(* Logix 5000 AddOnInstructionDefinition export Banner_B25_B55_Param_v4; software revision 33.00 *)

TYPE Banner_B25_B55_Configuration_v4 :
STRUCT
   Sensor_Lockout : SINT;   // 0=Unlocked, 1=Locked
   Sensitivity : SINT;   // 0=Low, 1=Standard, 2=High
   Pin2_Function : SINT;   // 0=Disabled, 1=Remote Teach, 2=Detection Output, 3=Complementary Output, 4=NC Health, 5=NO Health
   Pin2_Pin4_Polarity : SINT;   // 0=NPN, 1=PNP, 2=Push Pull
   Output_Logic : SINT;   // 0=LO, 1= DO
   Output_Delay_Mode : SINT;   // 0=No Delay, 1=On/Off Delay
   Output_On_Delay : DINT;
   Output_Off_Delay : DINT;
   Dynamic_Teach_Timeout_Mode : SINT;   // 0=Cancel Teach, 1=Stop Teach
   Dynamic_Teach_Timeout_Duration : DINT;
   Alarm_Threshold : SINT;   // Set to 0% to disable alarm. Thresholds close to 100% will alarm near taught condition, thrsholds near 0% will alarm near sensor limits
   Display_Disable : SINT;   // 0=Enabled, 1=Disabled
   Drift_Filter_Enable : SINT;   // 0=Disabled, 1=Enabled
   Signal_Mode : SINT;   // Signal Mode - Signal places 100% at taught condition and 0% at no signal. Switchpoint Centric paces 100% at taught conditition and 50% at switchpoint.
END_STRUCT
END_TYPE

TYPE Banner_B25_B55_RD_v4 :   // UDT that stores the Read Data for a B25 or B55.
STRUCT
   Direct : Banner_Direct_Parameters_v4;
   Serial_Number : STRING;
   Teach_State : SINT;   // 0=Idle, 1=SP1 Success, 2=SP2 Succes, 3=SP1 SP2 Success, 4 = Wait for Command, 5 = Busy, 7 = Error.
   Status : Banner_B25_B55_Status_v4;
   All_Time_Run_Time_Counter : DINT;   // 0 to 2 Billion. 1/4 hr increments.
END_STRUCT
END_TYPE

TYPE Banner_B25_B55_Status_v4 :
STRUCT
   Output_State : SINT;   // 0=Inactive, 1=Active
   Signal_Level : SINT;   // Signal Level - Switchpoit is at 50%, Taught Signal is at 100%
   Temperature : DINT;   // Internal Temperature
   Last_Taught_Temperature : DINT;   // Internal Temperature the last time device was taught
   Quality_of_Teach : SINT;   // 0=Not Taught, 1=Good, 2=Bad
   Health_Alarm_State : SINT;   // 0=No Alarm, 1= Alarm
   Quality_of_Health : INT;
END_STRUCT
END_TYPE

TYPE Banner_B25_B55_v4 :   // All of the parameters for a B25 or B55.
STRUCT
   Initial_Global_Read : BOOL;   // Determines if all of the IO-Link data has been read into the PLC yet
   Command : INT;   // Value placed in here will activate a read or write to a specifc IO-Link Index
   Read : Banner_B25_B55_RD_v4;   // Read Only Data
   Write : Banner_B25_B55_WD_v4;   // Write Data
   Reset : BOOL;   // Resets AOI. This will force a complete parameter read of the sensor.
END_STRUCT
END_TYPE

TYPE Banner_B25_B55_WD_v4 :   // UDT that stores the Write Data for a B25 or B55.
STRUCT
   System_Command : INT;   // See IODD file for list of commands that can be activated via the System Command interface
   Parameter_Access_Lock : SINT;   // Write access to all parameters is prohibited while value is 1. Only this parameter can be adjusted when value is 1.
   Data_Storage_Lock : SINT;   // Automatic data storage is disabled when this value is equal to 1. Read access is not affected.
   Local_Parameterization_Lock : SINT;   // Parameterization via local control elements on device is disabled.
   Local_User_Interface_Lock : SINT;   // Operation of local user interface is disabled.
   Configuration : Banner_B25_B55_Configuration_v4;
   Resettable_Run_Time_Counter : DINT;   // 0 to 2 Billion. 1/4 hr increments.
   All_Time_Run_Time_Event_Time : DINT;   // 0 to 2 Billion. 1/4 hr increments.
   Resettable_Run_Time_Event_Time_Counter : DINT;   // 0 to 2 Billion. 1/4 hr increments.
END_STRUCT
END_TYPE

TYPE Banner_Direct_Parameters_v4 :
STRUCT
   Master_Cycle_Time : INT;
   Min_Cycle_Time : INT;
   M_Sequence_Capability : INT;
   IO_Link_Version_ID : INT;
   Process_Data_Input_Length : INT;
   Process_Data_Output_Length : INT;
   Combined_Vendor_ID : DINT;   // IO-Link Vendor ID
   Vendor_ID1 : INT;
   Vendor_ID2 : INT;
   Combined_Device_ID : DINT;   // IO-Link Device ID
   Device_ID1 : INT;
   Device_ID2 : INT;
   Device_ID3 : INT;
END_STRUCT
END_TYPE

TYPE Banner_IOL_Port_v4 :   // UDT that has all of the data items necessary to communicate with a specific Port on a IO-Link Master
STRUCT
   Port_Controlled : INT;   // Each bit represents a port on an IO-Link Master. Set to 1 to tell AOI to control that port.
   Port_Activate : INT;   // Each bit represents a port on an IO-Link Master. When ON that port will process any commands in queue.
   Port_Read : INT;   // Each bit represents a port on an IO-Link Master. Used to determine when device AOI has requested a Read command.
   Port_Write : INT;   // Each bit represents a port on an IO-Link Master. Used to determine when device AOI has requested a Write command.
   Port_RW_Complete : INT;   // Each bit represents a port on an IO-Link Master. Tells device AOI that Read or Write request has been completed.
   Port_Device_Read : INT;
   Data_Transfer : SINT[190];   // Array to transfer data from IO-Master to device AOIs.
END_STRUCT
END_TYPE

ADD_ON_INSTRUCTION Banner_B25_B55_Param_v4   (* revision 4.0, vendor Banner Engineering *)
// AOI to read and write parameter data to an IO-Link B25 or B55.
VAR_IN_OUT
   Device : Banner_B25_B55_v4; {required}
   Port_Data : Banner_IOL_Port_v4; {required}
END_VAR
VAR_INPUT
   Port : DINT; {required}
   Type : DINT; {required}
END_VAR
VAR
   Local_Control : DINT; {access None}
   Global_Read_Command_Value : INT; {access None}
   Global_Write_Command_Value : INT; {access None}
   Command_Being_Processed : BOOL; {access None}
   Update_Archive : BOOL; {access None}
   Index_Write_Inprocess : INT; {access None}
   Index_Write_Control : INT; {access None}
   Inprocess_Index : DINT; {access None}
END_VAR

ROUTINE Logic   (* ladder *)
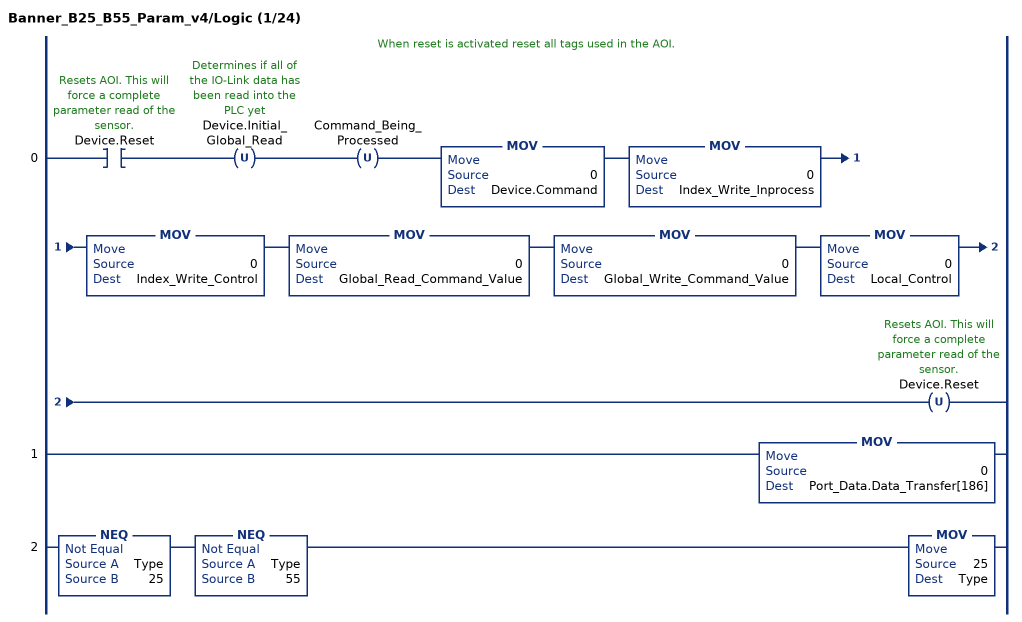
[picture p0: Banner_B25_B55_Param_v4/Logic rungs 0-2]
   // When reset is activated reset all tags used in the AOI.
   0: XIC(Device.Reset)OTU(Device.Initial_Global_Read)OTU(Command_Being_Processed)MOV(0,Device.Command)MOV(0,Index_Write_Inprocess)MOV(0,Index_Write_Control)MOV(0,Global_Read_Command_Value)MOV(0,Global_Write_Command_Value)MOV(0,Local_Control)OTU(Device.Reset);
   1: MOV(0,Port_Data.Data_Transfer[186]);
   2: NEQ(Type,25)NEQ(Type,55)MOV(25,Type);
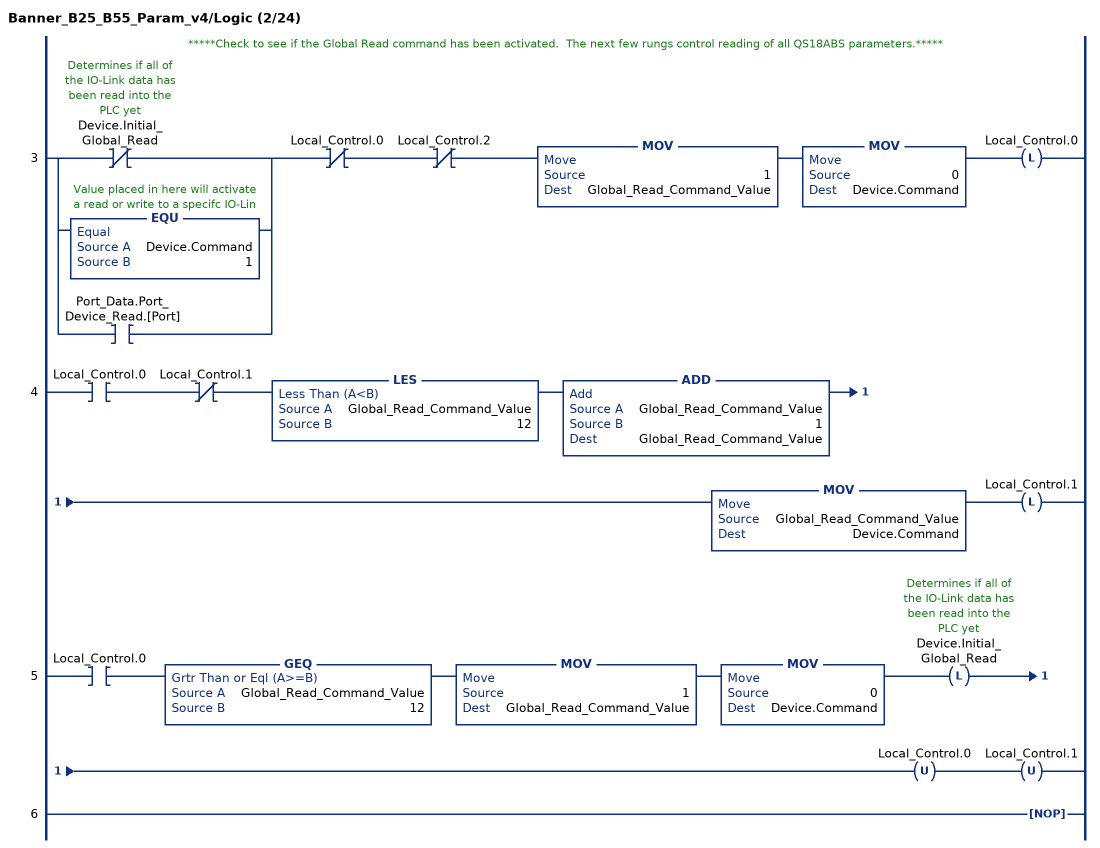
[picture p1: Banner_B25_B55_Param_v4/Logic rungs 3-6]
   // *****Check to see if the Global Read command has been activated.  The next few rungs control reading of all QS18ABS parameters.*****
   3: [XIO(Device.Initial_Global_Read) ,EQU(Device.Command,1) ,XIC(Port_Data.Port_Device_Read.[Port]) ]XIO(Local_Control.0)XIO(Local_Control.2)MOV(1,Global_Read_Command_Value)MOV(0,Device.Command)OTL(Local_Control.0);
   4: XIC(Local_Control.0)XIO(Local_Control.1)LES(Global_Read_Command_Value,12)ADD(Global_Read_Command_Value,1,Global_Read_Command_Value)MOV(Global_Read_Command_Value,Device.Command)OTL(Local_Control.1);
   5: XIC(Local_Control.0)GEQ(Global_Read_Command_Value,12)MOV(1,Global_Read_Command_Value)MOV(0,Device.Command)OTL(Device.Initial_Global_Read)OTU(Local_Control.0)OTU(Local_Control.1);
   6: NOP();
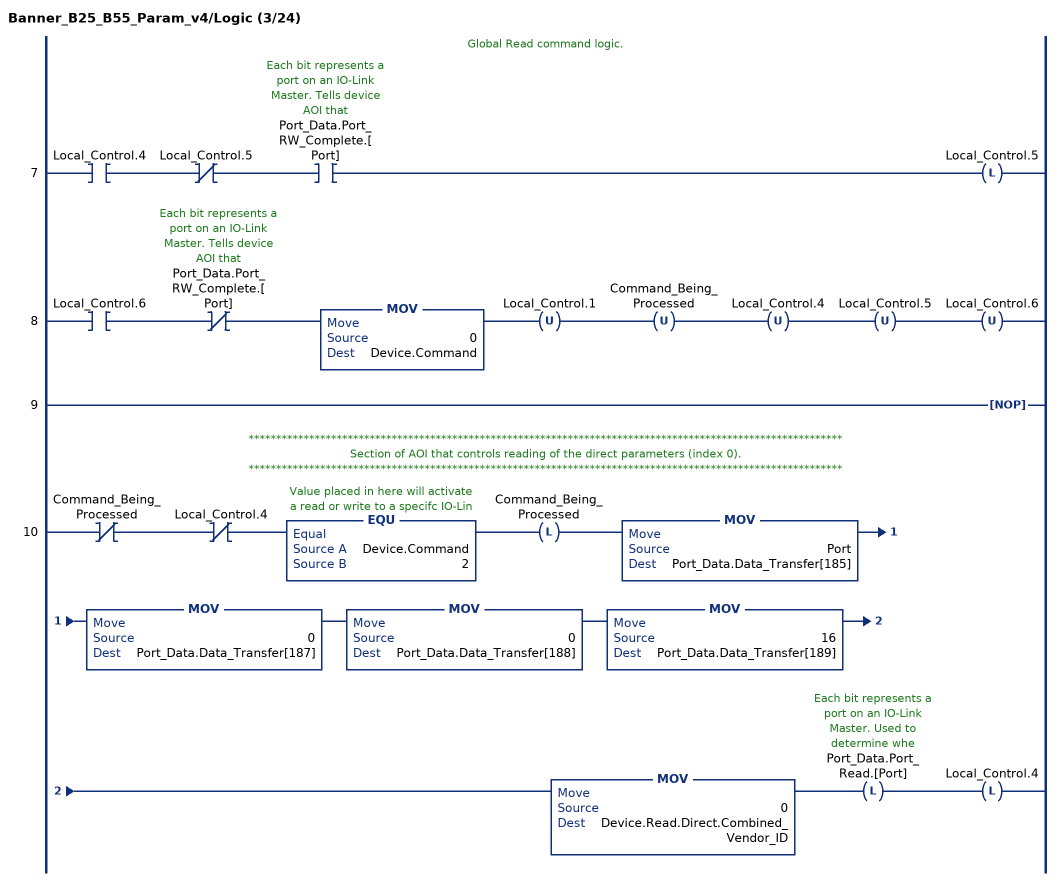
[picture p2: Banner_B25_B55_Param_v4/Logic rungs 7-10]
   // Global Read command logic.
   7: XIC(Local_Control.4)XIO(Local_Control.5)XIC(Port_Data.Port_RW_Complete.[Port])OTL(Local_Control.5);
   8: XIC(Local_Control.6)XIO(Port_Data.Port_RW_Complete.[Port])MOV(0,Device.Command)OTU(Local_Control.1)OTU(Command_Being_Processed)OTU(Local_Control.4)OTU(Local_Control.5)OTU(Local_Control.6);
   9: NOP();
   // ************************************************************************************************************
   // Section of AOI that controls reading of the direct parameters (index 0).
   // ************************************************************************************************************
   10: XIO(Command_Being_Processed)XIO(Local_Control.4)EQU(Device.Command,2)OTL(Command_Being_Processed)MOV(Port,Port_Data.Data_Transfer[185])MOV(0,Port_Data.Data_Transfer[187])MOV(0,Port_Data.Data_Transfer[188])MOV(16,Port_Data.Data_Transfer[189])MOV(0,Device.Read.Direct.Combined_Vendor_ID)OTL(Port_Data.Port_Read.[Port])OTL(Local_Control.4);
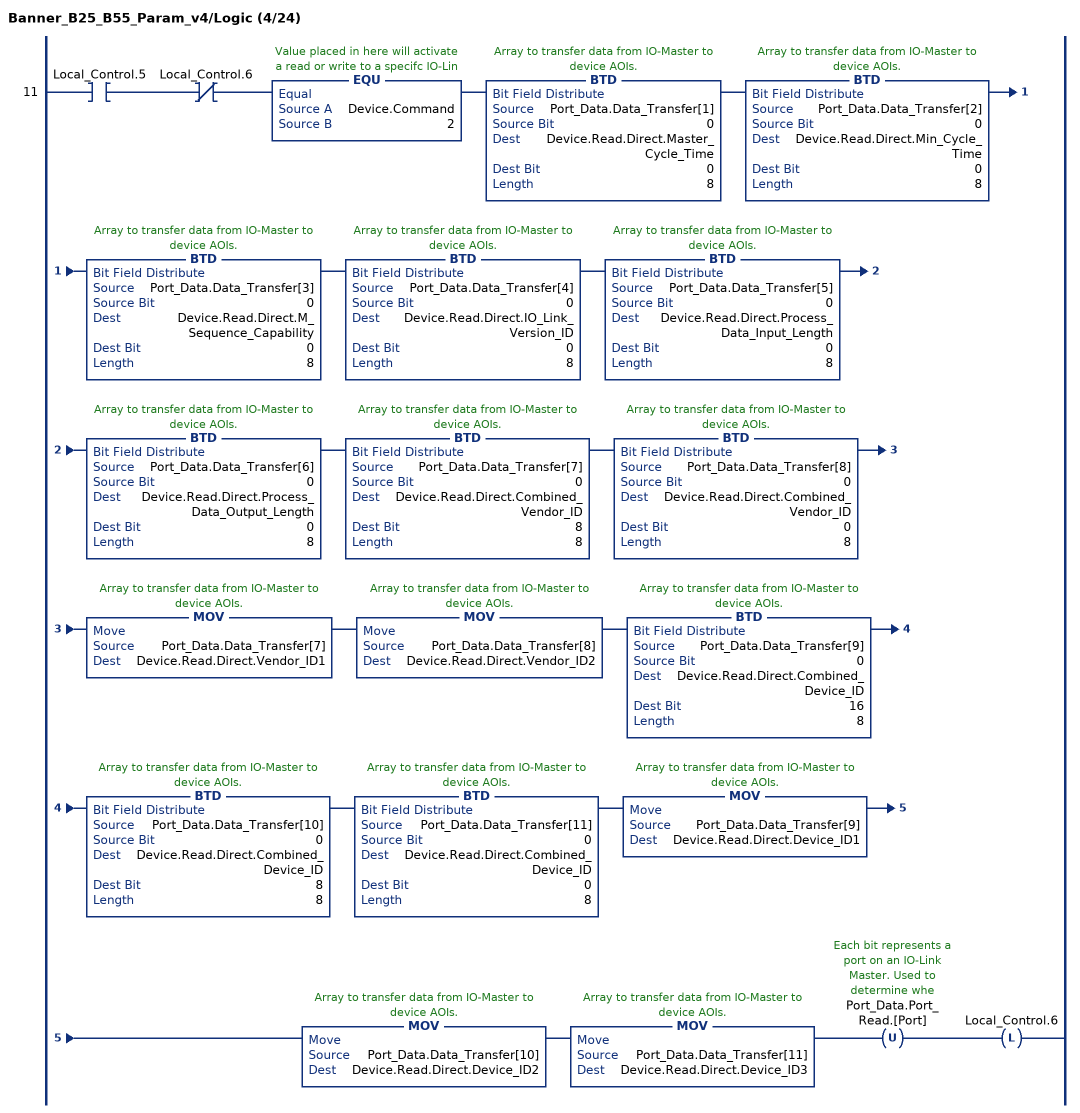
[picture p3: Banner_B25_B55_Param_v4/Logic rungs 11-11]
   11: XIC(Local_Control.5)XIO(Local_Control.6)EQU(Device.Command,2)BTD(Port_Data.Data_Transfer[1],0,Device.Read.Direct.Master_Cycle_Time,0,8)BTD(Port_Data.Data_Transfer[2],0,Device.Read.Direct.Min_Cycle_Time,0,8)BTD(Port_Data.Data_Transfer[3],0,Device.Read.Direct.M_Sequence_Capability,0,8)BTD(Port_Data.Data_Transfer[4],0,Device.Read.Direct.IO_Link_Version_ID,0,8)BTD(Port_Data.Data_Transfer[5],0,Device.Read.Direct.Process_Data_Input_Length,0,8)BTD(Port_Data.Data_Transfer[6],0,Device.Read.Direct.Process_Data_Output_Length,0,8)BTD(Port_Data.Data_Transfer[7],0,Device.Read.Direct.Combined_Vendor_ID,8,8)BTD(Port_Data.Data_Transfer[8],0,Device.Read.Direct.Combined_Vendor_ID,0,8)MOV(Port_Data.Data_Transfer[7],Device.Read.Direct.Vendor_ID1)MOV(Port_Data.Data_Transfer[8],Device.Read.Direct.Vendor_ID2)BTD(Port_Data.Data_Transfer[9],0,Device.Read.Direct.Combined_Device_ID,16,8)BTD(Port_Data.Data_Transfer[10],0,Device.Read.Direct.Combined_Device_ID,8,8)BTD(Port_Data.Data_Transfer[11],0,Device.Read.Direct.Combined_Device_ID,0,8)MOV(Port_Data.Data_Transfer[9],Device.Read.Direct.Device_ID1)MOV(Port_Data.Data_Transfer[10],Device.Read.Direct.Device_ID2)MOV(Port_Data.Data_Transfer[11],Device.Read.Direct.Device_ID3)OTU(Port_Data.Port_Read.[Port])OTL(Local_Control.6);
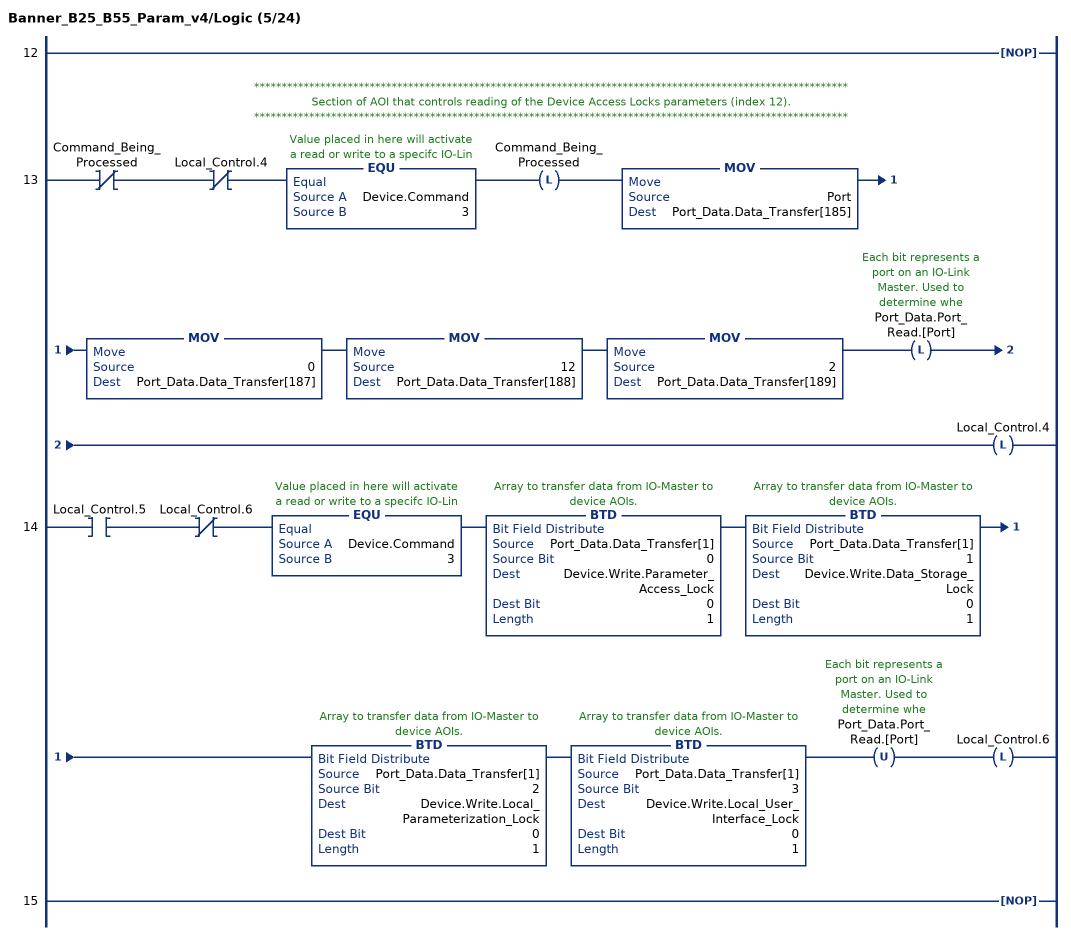
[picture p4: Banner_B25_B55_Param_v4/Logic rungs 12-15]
   12: NOP();
   // ************************************************************************************************************
   // Section of AOI that controls reading of the Device Access Locks parameters (index 12).
   // ************************************************************************************************************
   13: XIO(Command_Being_Processed)XIO(Local_Control.4)EQU(Device.Command,3)OTL(Command_Being_Processed)MOV(Port,Port_Data.Data_Transfer[185])MOV(0,Port_Data.Data_Transfer[187])MOV(12,Port_Data.Data_Transfer[188])MOV(2,Port_Data.Data_Transfer[189])OTL(Port_Data.Port_Read.[Port])OTL(Local_Control.4);
   14: XIC(Local_Control.5)XIO(Local_Control.6)EQU(Device.Command,3)BTD(Port_Data.Data_Transfer[1],0,Device.Write.Parameter_Access_Lock,0,1)BTD(Port_Data.Data_Transfer[1],1,Device.Write.Data_Storage_Lock,0,1)BTD(Port_Data.Data_Transfer[1],2,Device.Write.Local_Parameterization_Lock,0,1)BTD(Port_Data.Data_Transfer[1],3,Device.Write.Local_User_Interface_Lock,0,1)OTU(Port_Data.Port_Read.[Port])OTL(Local_Control.6);
   15: NOP();
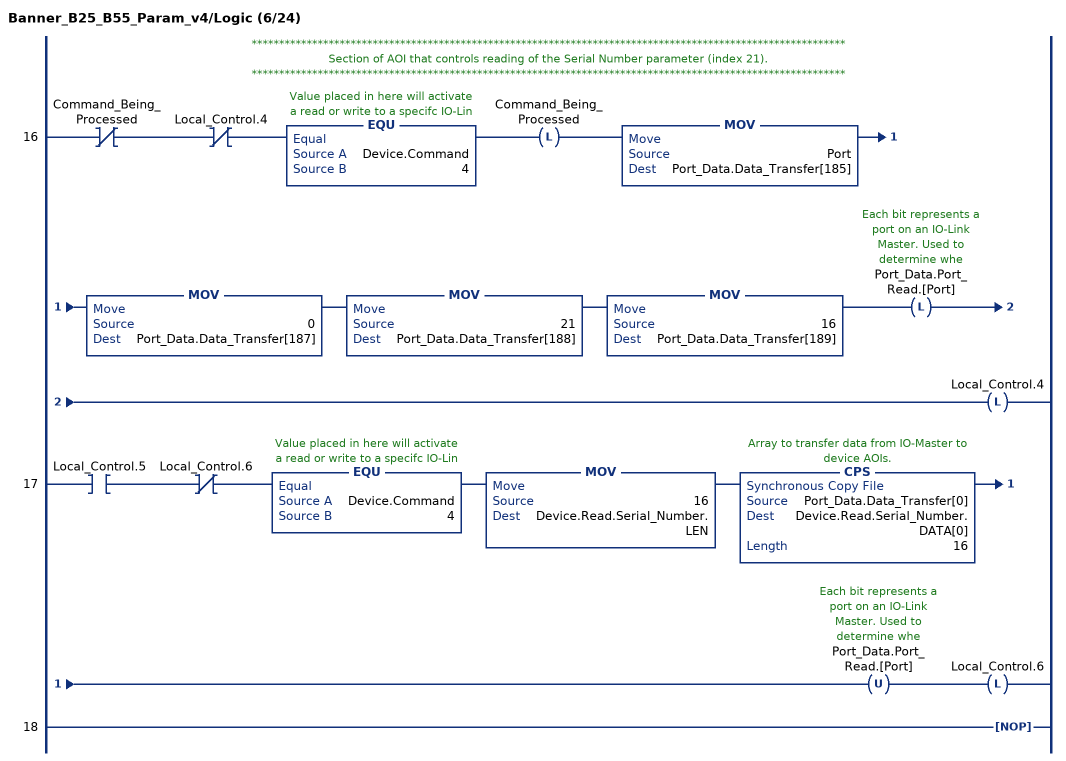
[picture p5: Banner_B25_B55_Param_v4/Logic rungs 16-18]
   // ************************************************************************************************************
   // Section of AOI that controls reading of the Serial Number parameter (index 21).
   // ************************************************************************************************************
   16: XIO(Command_Being_Processed)XIO(Local_Control.4)EQU(Device.Command,4)OTL(Command_Being_Processed)MOV(Port,Port_Data.Data_Transfer[185])MOV(0,Port_Data.Data_Transfer[187])MOV(21,Port_Data.Data_Transfer[188])MOV(16,Port_Data.Data_Transfer[189])OTL(Port_Data.Port_Read.[Port])OTL(Local_Control.4);
   17: XIC(Local_Control.5)XIO(Local_Control.6)EQU(Device.Command,4)MOV(16,Device.Read.Serial_Number.LEN)CPS(Port_Data.Data_Transfer[0],Device.Read.Serial_Number.DATA[0],16)OTU(Port_Data.Port_Read.[Port])OTL(Local_Control.6);
   18: NOP();
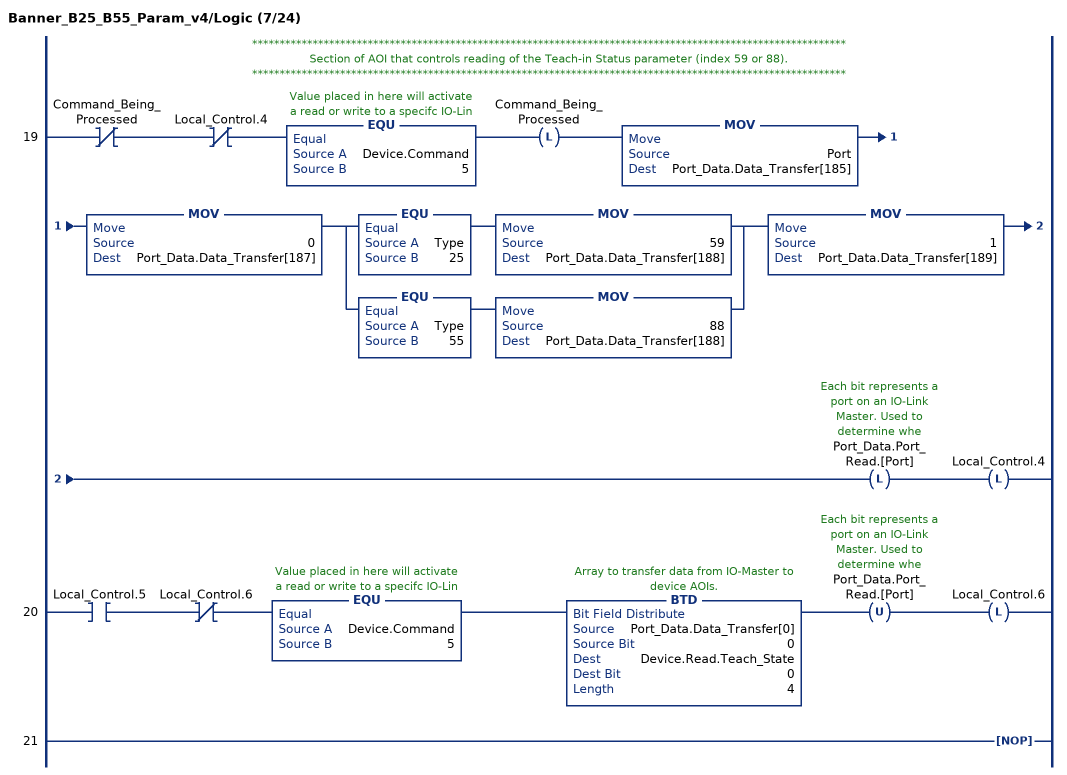
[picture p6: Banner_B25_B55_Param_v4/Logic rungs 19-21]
   // ************************************************************************************************************
   // Section of AOI that controls reading of the Teach-in Status parameter (index 59 or 88).
   // ************************************************************************************************************
   19: XIO(Command_Being_Processed)XIO(Local_Control.4)EQU(Device.Command,5)OTL(Command_Being_Processed)MOV(Port,Port_Data.Data_Transfer[185])MOV(0,Port_Data.Data_Transfer[187])[EQU(Type,25) MOV(59,Port_Data.Data_Transfer[188]) ,EQU(Type,55) MOV(88,Port_Data.Data_Transfer[188]) ]MOV(1,Port_Data.Data_Transfer[189])OTL(Port_Data.Port_Read.[Port])OTL(Local_Control.4);
   20: XIC(Local_Control.5)XIO(Local_Control.6)EQU(Device.Command,5)BTD(Port_Data.Data_Transfer[0],0,Device.Read.Teach_State,0,4)OTU(Port_Data.Port_Read.[Port])OTL(Local_Control.6);
   21: NOP();
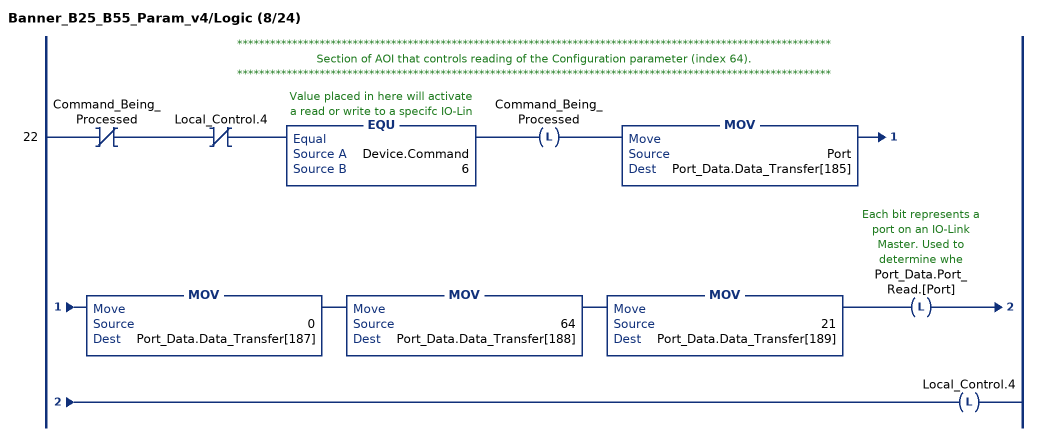
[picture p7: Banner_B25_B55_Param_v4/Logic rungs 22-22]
   // ************************************************************************************************************
   // Section of AOI that controls reading of the Configuration parameter (index 64).
   // ************************************************************************************************************
   22: XIO(Command_Being_Processed)XIO(Local_Control.4)EQU(Device.Command,6)OTL(Command_Being_Processed)MOV(Port,Port_Data.Data_Transfer[185])MOV(0,Port_Data.Data_Transfer[187])MOV(64,Port_Data.Data_Transfer[188])MOV(21,Port_Data.Data_Transfer[189])OTL(Port_Data.Port_Read.[Port])OTL(Local_Control.4);
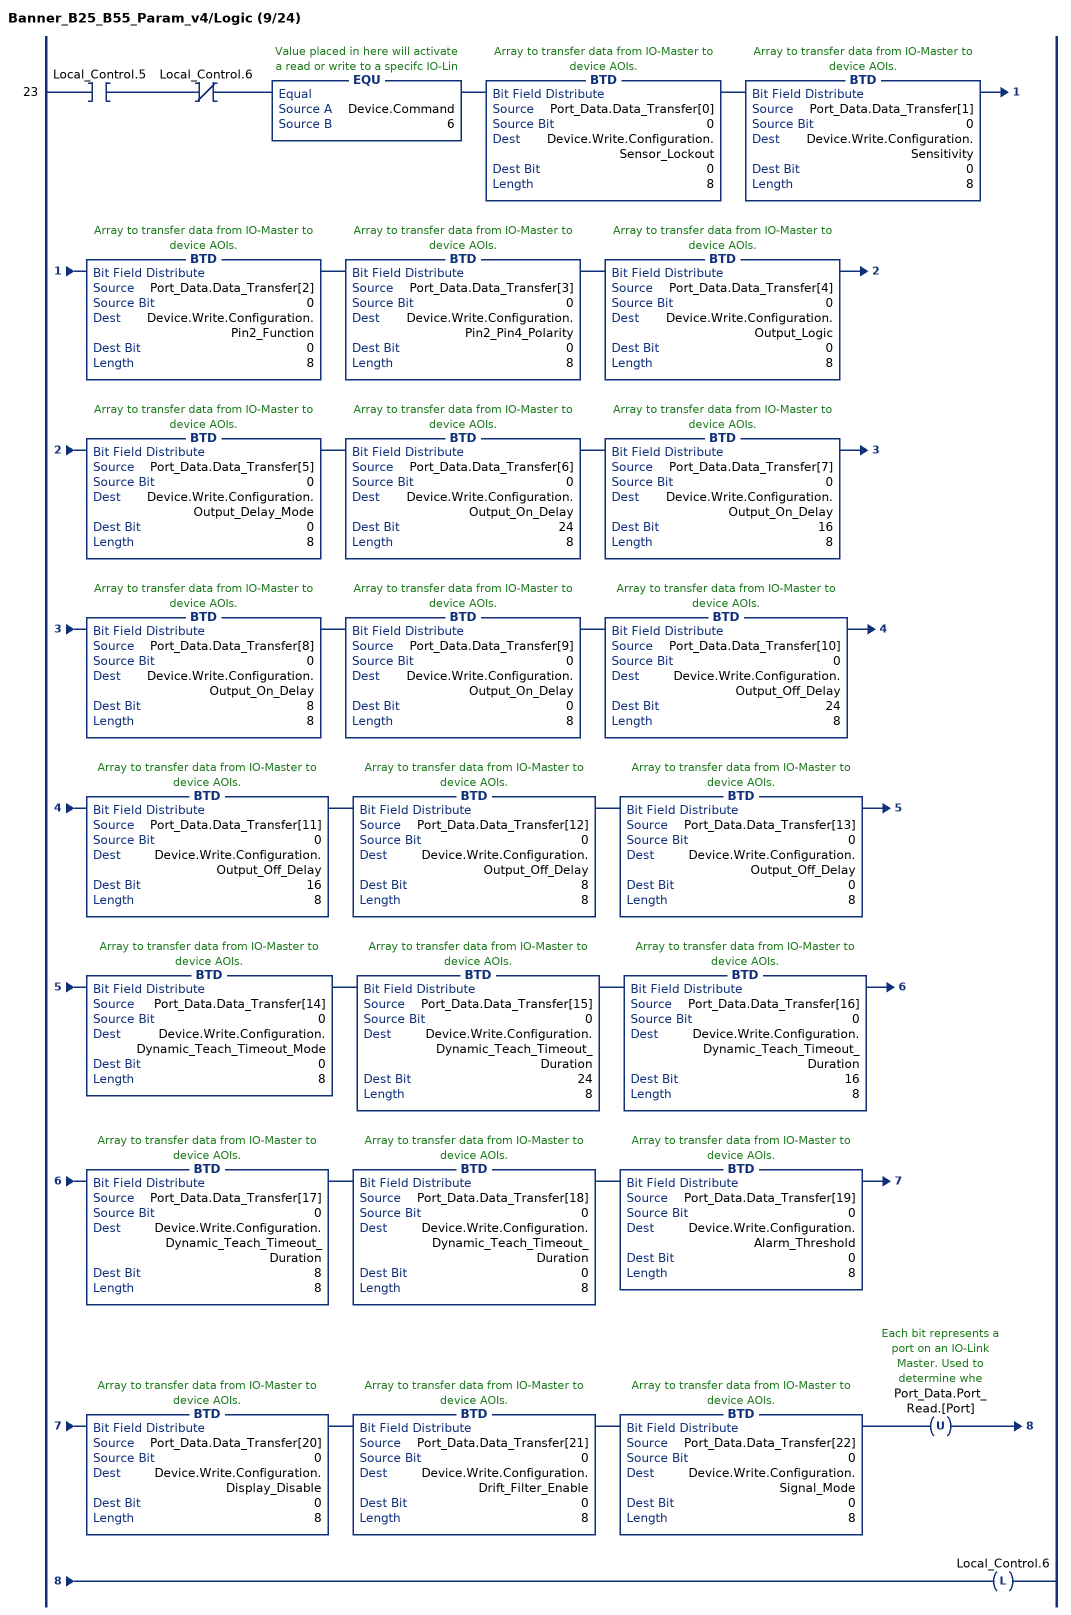
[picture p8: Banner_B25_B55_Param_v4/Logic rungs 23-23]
   23: XIC(Local_Control.5)XIO(Local_Control.6)EQU(Device.Command,6)BTD(Port_Data.Data_Transfer[0],0,Device.Write.Configuration.Sensor_Lockout,0,8)BTD(Port_Data.Data_Transfer[1],0,Device.Write.Configuration.Sensitivity,0,8)BTD(Port_Data.Data_Transfer[2],0,Device.Write.Configuration.Pin2_Function,0,8)BTD(Port_Data.Data_Transfer[3],0,Device.Write.Configuration.Pin2_Pin4_Polarity,0,8)BTD(Port_Data.Data_Transfer[4],0,Device.Write.Configuration.Output_Logic,0,8)BTD(Port_Data.Data_Transfer[5],0,Device.Write.Configuration.Output_Delay_Mode,0,8)BTD(Port_Data.Data_Transfer[6],0,Device.Write.Configuration.Output_On_Delay,24,8)BTD(Port_Data.Data_Transfer[7],0,Device.Write.Configuration.Output_On_Delay,16,8)BTD(Port_Data.Data_Transfer[8],0,Device.Write.Configuration.Output_On_Delay,8,8)BTD(Port_Data.Data_Transfer[9],0,Device.Write.Configuration.Output_On_Delay,0,8)BTD(Port_Data.Data_Transfer[10],0,Device.Write.Configuration.Output_Off_Delay,24,8)BTD(Port_Data.Data_Transfer[11],0,Device.Write.Configuration.Output_Off_Delay,16,8)BTD(Port_Data.Data_Transfer[12],0,Device.Write.Configuration.Output_Off_Delay,8,8)BTD(Port_Data.Data_Transfer[13],0,Device.Write.Configuration.Output_Off_Delay,0,8)BTD(Port_Data.Data_Transfer[14],0,Device.Write.Configuration.Dynamic_Teach_Timeout_Mode,0,8)BTD(Port_Data.Data_Transfer[15],0,Device.Write.Configuration.Dynamic_Teach_Timeout_Duration,24,8)BTD(Port_Data.Data_Transfer[16],0,Device.Write.Configuration.Dynamic_Teach_Timeout_Duration,16,8)BTD(Port_Data.Data_Transfer[17],0,Device.Write.Configuration.Dynamic_Teach_Timeout_Duration,8,8)BTD(Port_Data.Data_Transfer[18],0,Device.Write.Configuration.Dynamic_Teach_Timeout_Duration,0,8)BTD(Port_Data.Data_Transfer[19],0,Device.Write.Configuration.Alarm_Threshold,0,8)BTD(Port_Data.Data_Transfer[20],0,Device.Write.Configuration.Display_Disable,0,8)BTD(Port_Data.Data_Transfer[21],0,Device.Write.Configuration.Drift_Filter_Enable,0,8)BTD(Port_Data.Data_Transfer[22],0,Device.Write.Configuration.Signal_Mode,0,8)OTU(Port_Data.Port_Read.[Port])OTL(Local_Control.6);
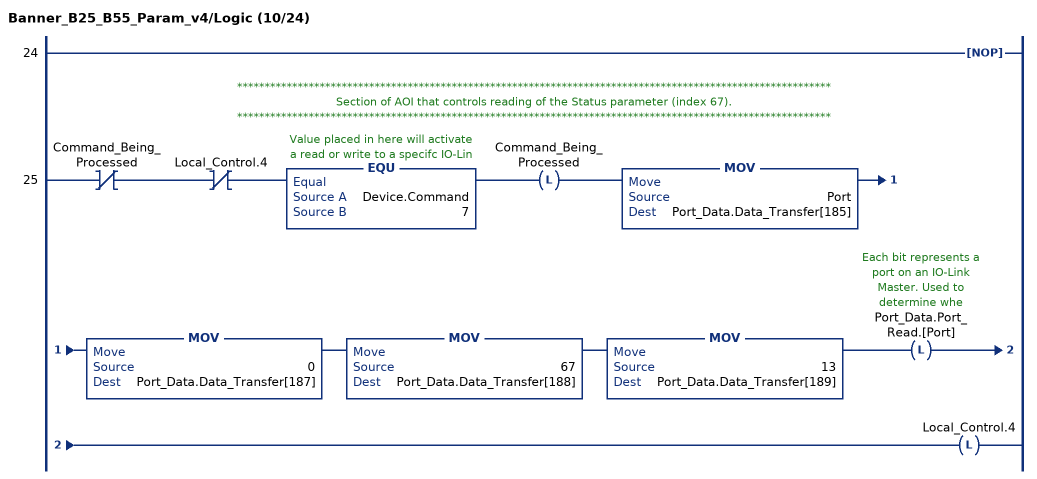
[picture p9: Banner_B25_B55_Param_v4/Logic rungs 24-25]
   24: NOP();
   // ************************************************************************************************************
   // Section of AOI that controls reading of the Status parameter (index 67).
   // ************************************************************************************************************
   25: XIO(Command_Being_Processed)XIO(Local_Control.4)EQU(Device.Command,7)OTL(Command_Being_Processed)MOV(Port,Port_Data.Data_Transfer[185])MOV(0,Port_Data.Data_Transfer[187])MOV(67,Port_Data.Data_Transfer[188])MOV(13,Port_Data.Data_Transfer[189])OTL(Port_Data.Port_Read.[Port])OTL(Local_Control.4);
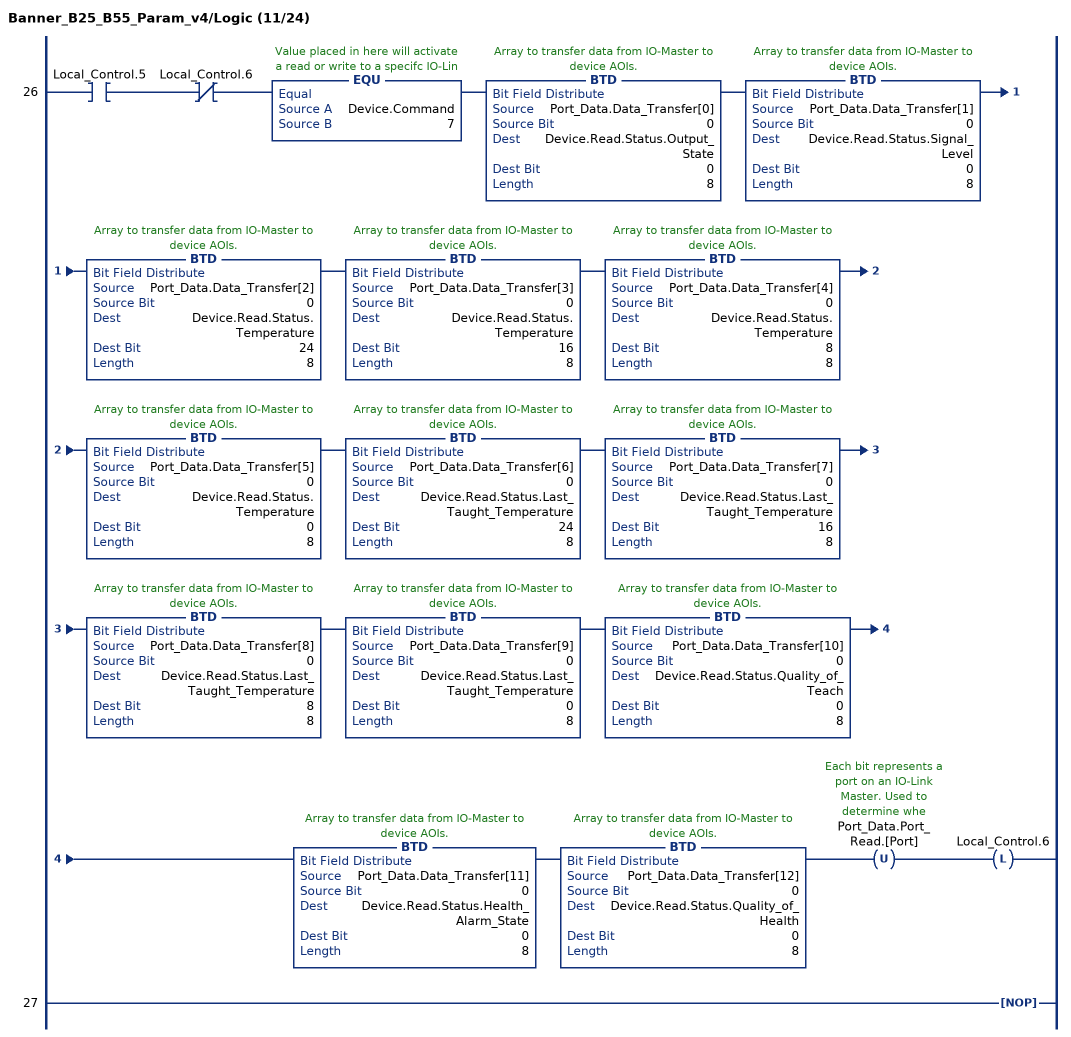
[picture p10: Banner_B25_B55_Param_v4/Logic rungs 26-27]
   26: XIC(Local_Control.5)XIO(Local_Control.6)EQU(Device.Command,7)BTD(Port_Data.Data_Transfer[0],0,Device.Read.Status.Output_State,0,8)BTD(Port_Data.Data_Transfer[1],0,Device.Read.Status.Signal_Level,0,8)BTD(Port_Data.Data_Transfer[2],0,Device.Read.Status.Temperature,24,8)BTD(Port_Data.Data_Transfer[3],0,Device.Read.Status.Temperature,16,8)BTD(Port_Data.Data_Transfer[4],0,Device.Read.Status.Temperature,8,8)BTD(Port_Data.Data_Transfer[5],0,Device.Read.Status.Temperature,0,8)BTD(Port_Data.Data_Transfer[6],0,Device.Read.Status.Last_Taught_Temperature,24,8)BTD(Port_Data.Data_Transfer[7],0,Device.Read.Status.Last_Taught_Temperature,16,8)BTD(Port_Data.Data_Transfer[8],0,Device.Read.Status.Last_Taught_Temperature,8,8)BTD(Port_Data.Data_Transfer[9],0,Device.Read.Status.Last_Taught_Temperature,0,8)BTD(Port_Data.Data_Transfer[10],0,Device.Read.Status.Quality_of_Teach,0,8)BTD(Port_Data.Data_Transfer[11],0,Device.Read.Status.Health_Alarm_State,0,8)BTD(Port_Data.Data_Transfer[12],0,Device.Read.Status.Quality_of_Health,0,8)OTU(Port_Data.Port_Read.[Port])OTL(Local_Control.6);
   27: NOP();
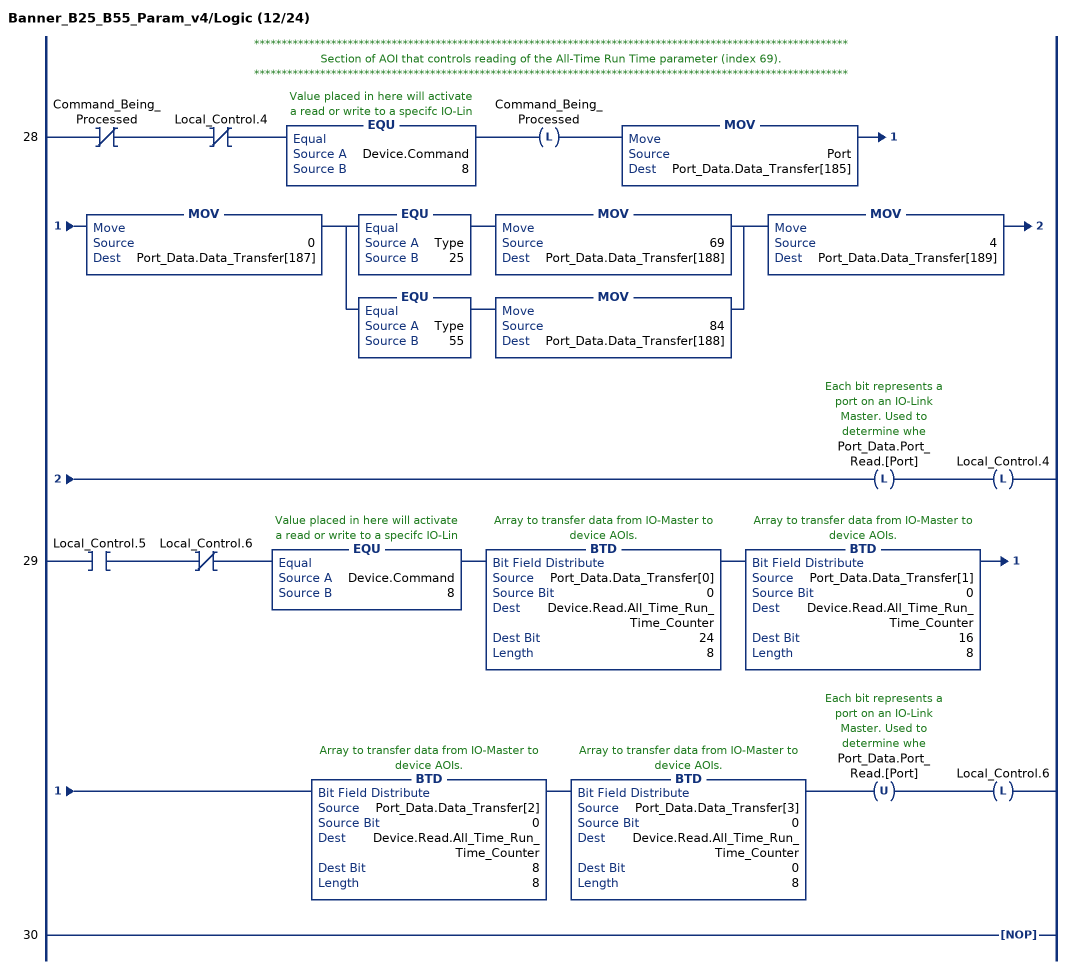
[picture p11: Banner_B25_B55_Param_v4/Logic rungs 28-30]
   // ************************************************************************************************************
   // Section of AOI that controls reading of the All-Time Run Time parameter (index 69).
   // ************************************************************************************************************
   28: XIO(Command_Being_Processed)XIO(Local_Control.4)EQU(Device.Command,8)OTL(Command_Being_Processed)MOV(Port,Port_Data.Data_Transfer[185])MOV(0,Port_Data.Data_Transfer[187])[EQU(Type,25) MOV(69,Port_Data.Data_Transfer[188]) ,EQU(Type,55) MOV(84,Port_Data.Data_Transfer[188]) ]MOV(4,Port_Data.Data_Transfer[189])OTL(Port_Data.Port_Read.[Port])OTL(Local_Control.4);
   29: XIC(Local_Control.5)XIO(Local_Control.6)EQU(Device.Command,8)BTD(Port_Data.Data_Transfer[0],0,Device.Read.All_Time_Run_Time_Counter,24,8)BTD(Port_Data.Data_Transfer[1],0,Device.Read.All_Time_Run_Time_Counter,16,8)BTD(Port_Data.Data_Transfer[2],0,Device.Read.All_Time_Run_Time_Counter,8,8)BTD(Port_Data.Data_Transfer[3],0,Device.Read.All_Time_Run_Time_Counter,0,8)OTU(Port_Data.Port_Read.[Port])OTL(Local_Control.6);
   30: NOP();
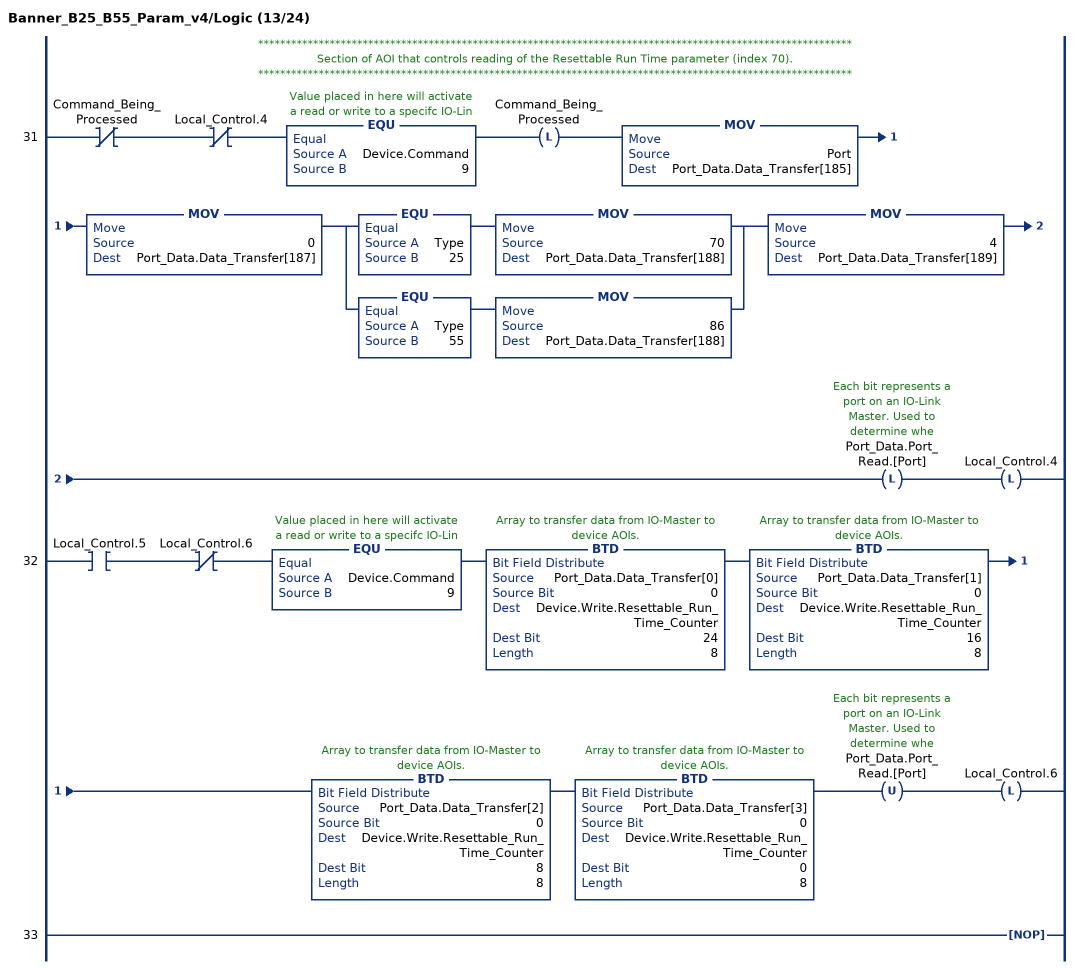
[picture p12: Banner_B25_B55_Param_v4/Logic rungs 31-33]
   // ************************************************************************************************************
   // Section of AOI that controls reading of the Resettable Run Time parameter (index 70).
   // ************************************************************************************************************
   31: XIO(Command_Being_Processed)XIO(Local_Control.4)EQU(Device.Command,9)OTL(Command_Being_Processed)MOV(Port,Port_Data.Data_Transfer[185])MOV(0,Port_Data.Data_Transfer[187])[EQU(Type,25) MOV(70,Port_Data.Data_Transfer[188]) ,EQU(Type,55) MOV(86,Port_Data.Data_Transfer[188]) ]MOV(4,Port_Data.Data_Transfer[189])OTL(Port_Data.Port_Read.[Port])OTL(Local_Control.4);
   32: XIC(Local_Control.5)XIO(Local_Control.6)EQU(Device.Command,9)BTD(Port_Data.Data_Transfer[0],0,Device.Write.Resettable_Run_Time_Counter,24,8)BTD(Port_Data.Data_Transfer[1],0,Device.Write.Resettable_Run_Time_Counter,16,8)BTD(Port_Data.Data_Transfer[2],0,Device.Write.Resettable_Run_Time_Counter,8,8)BTD(Port_Data.Data_Transfer[3],0,Device.Write.Resettable_Run_Time_Counter,0,8)OTU(Port_Data.Port_Read.[Port])OTL(Local_Control.6);
   33: NOP();
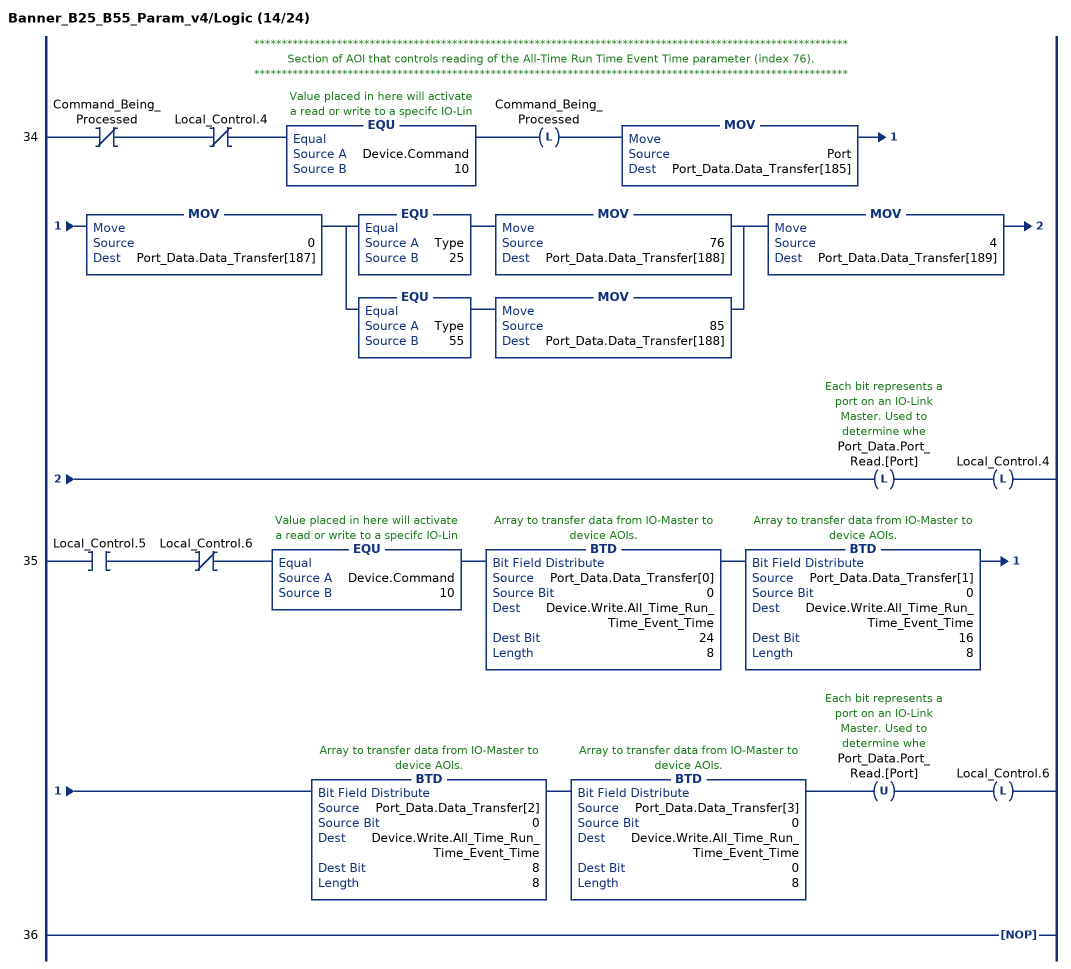
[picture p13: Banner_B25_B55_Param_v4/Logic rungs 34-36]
   // ************************************************************************************************************
   // Section of AOI that controls reading of the All-Time Run Time Event Time parameter (index 76).
   // ************************************************************************************************************
   34: XIO(Command_Being_Processed)XIO(Local_Control.4)EQU(Device.Command,10)OTL(Command_Being_Processed)MOV(Port,Port_Data.Data_Transfer[185])MOV(0,Port_Data.Data_Transfer[187])[EQU(Type,25) MOV(76,Port_Data.Data_Transfer[188]) ,EQU(Type,55) MOV(85,Port_Data.Data_Transfer[188]) ]MOV(4,Port_Data.Data_Transfer[189])OTL(Port_Data.Port_Read.[Port])OTL(Local_Control.4);
   35: XIC(Local_Control.5)XIO(Local_Control.6)EQU(Device.Command,10)BTD(Port_Data.Data_Transfer[0],0,Device.Write.All_Time_Run_Time_Event_Time,24,8)BTD(Port_Data.Data_Transfer[1],0,Device.Write.All_Time_Run_Time_Event_Time,16,8)BTD(Port_Data.Data_Transfer[2],0,Device.Write.All_Time_Run_Time_Event_Time,8,8)BTD(Port_Data.Data_Transfer[3],0,Device.Write.All_Time_Run_Time_Event_Time,0,8)OTU(Port_Data.Port_Read.[Port])OTL(Local_Control.6);
   36: NOP();
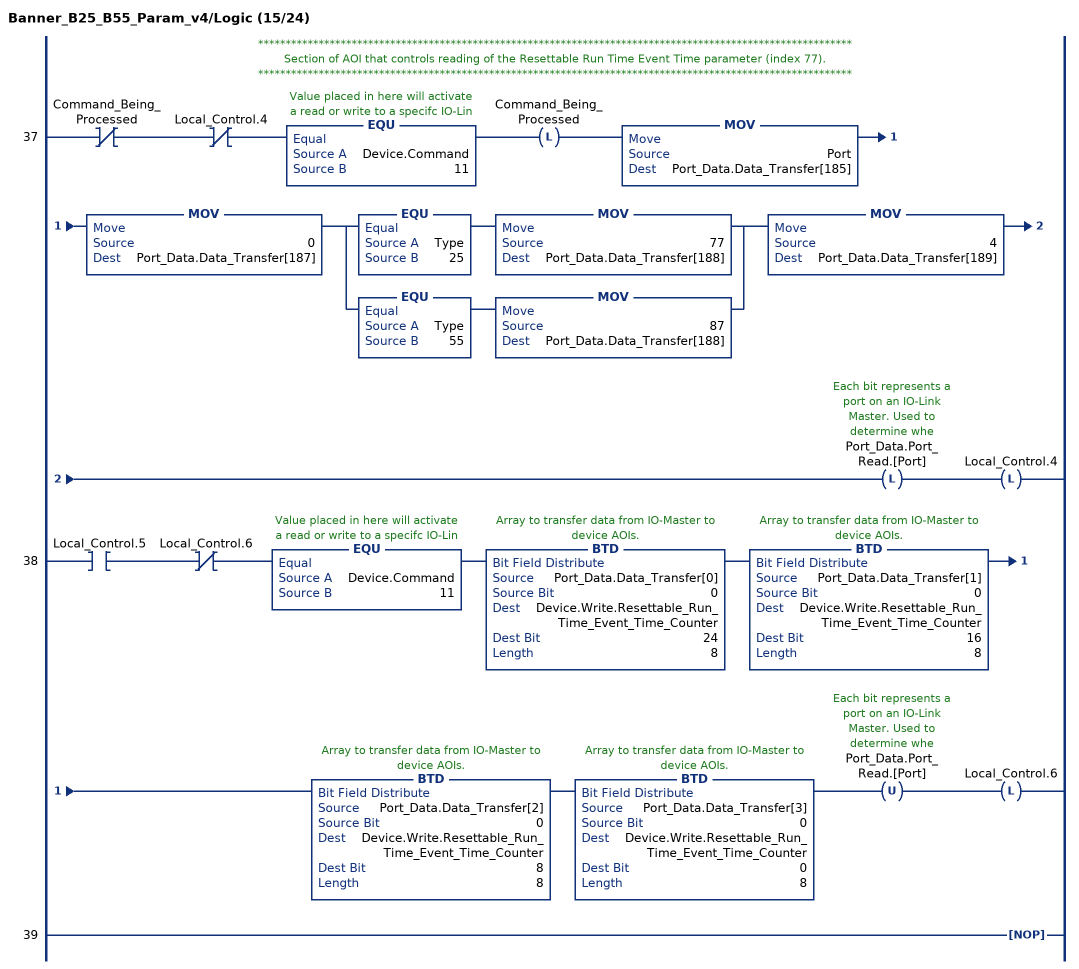
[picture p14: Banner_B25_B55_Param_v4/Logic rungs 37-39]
   // ************************************************************************************************************
   // Section of AOI that controls reading of the Resettable Run Time Event Time parameter (index 77).
   // ************************************************************************************************************
   37: XIO(Command_Being_Processed)XIO(Local_Control.4)EQU(Device.Command,11)OTL(Command_Being_Processed)MOV(Port,Port_Data.Data_Transfer[185])MOV(0,Port_Data.Data_Transfer[187])[EQU(Type,25) MOV(77,Port_Data.Data_Transfer[188]) ,EQU(Type,55) MOV(87,Port_Data.Data_Transfer[188]) ]MOV(4,Port_Data.Data_Transfer[189])OTL(Port_Data.Port_Read.[Port])OTL(Local_Control.4);
   38: XIC(Local_Control.5)XIO(Local_Control.6)EQU(Device.Command,11)BTD(Port_Data.Data_Transfer[0],0,Device.Write.Resettable_Run_Time_Event_Time_Counter,24,8)BTD(Port_Data.Data_Transfer[1],0,Device.Write.Resettable_Run_Time_Event_Time_Counter,16,8)BTD(Port_Data.Data_Transfer[2],0,Device.Write.Resettable_Run_Time_Event_Time_Counter,8,8)BTD(Port_Data.Data_Transfer[3],0,Device.Write.Resettable_Run_Time_Event_Time_Counter,0,8)OTU(Port_Data.Port_Read.[Port])OTL(Local_Control.6);
   39: NOP();
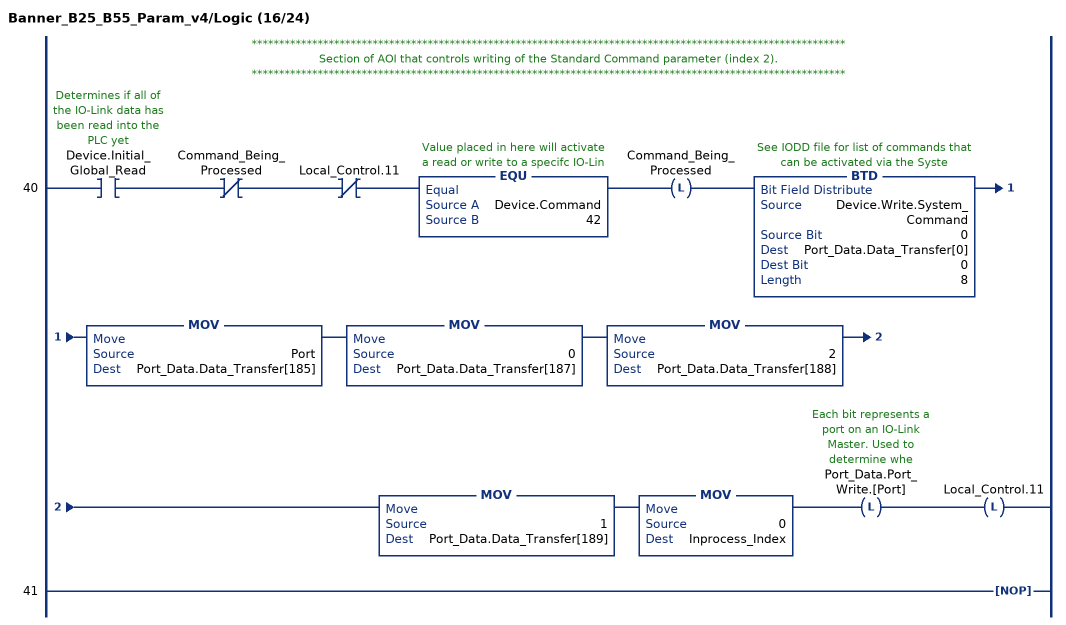
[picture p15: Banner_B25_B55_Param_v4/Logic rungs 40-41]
   // ************************************************************************************************************
   // Section of AOI that controls writing of the Standard Command parameter (index 2).
   // ************************************************************************************************************
   40: XIC(Device.Initial_Global_Read)XIO(Command_Being_Processed)XIO(Local_Control.11)EQU(Device.Command,42)OTL(Command_Being_Processed)BTD(Device.Write.System_Command,0,Port_Data.Data_Transfer[0],0,8)MOV(Port,Port_Data.Data_Transfer[185])MOV(0,Port_Data.Data_Transfer[187])MOV(2,Port_Data.Data_Transfer[188])MOV(1,Port_Data.Data_Transfer[189])MOV(0,Inprocess_Index)OTL(Port_Data.Port_Write.[Port])OTL(Local_Control.11);
   41: NOP();
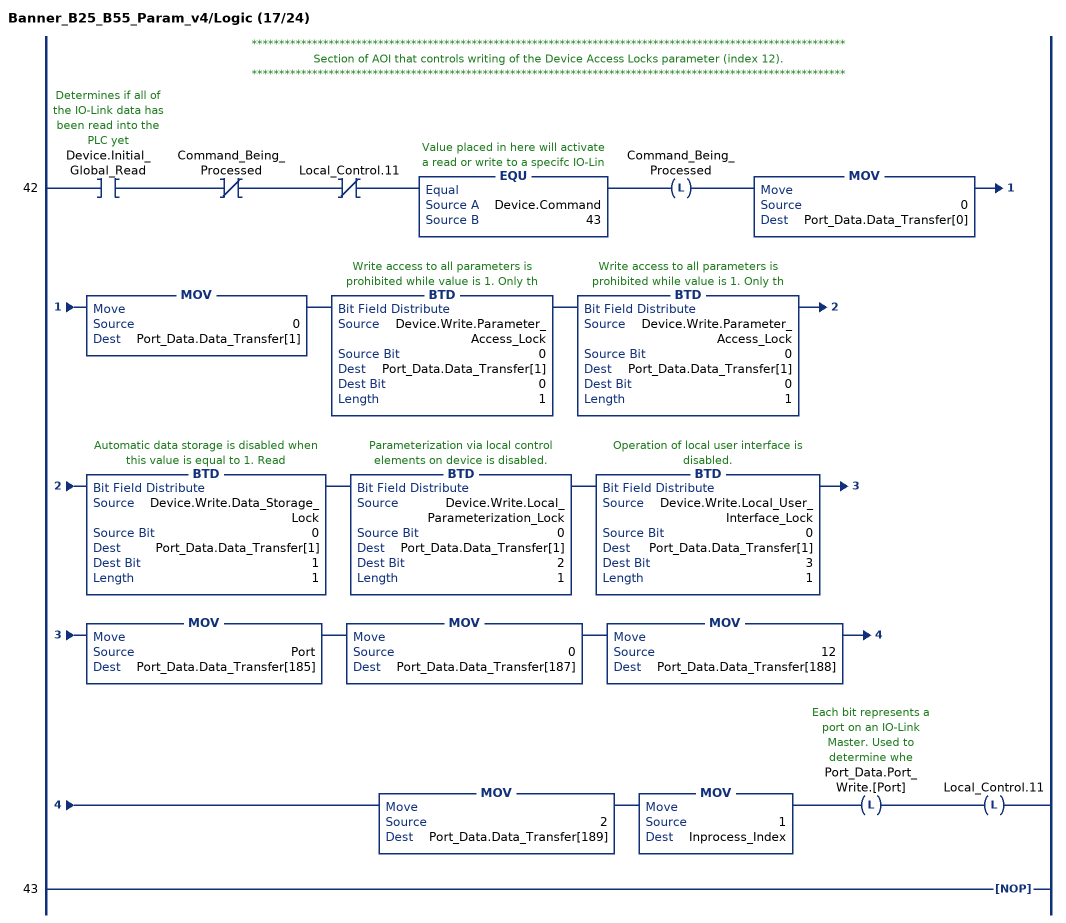
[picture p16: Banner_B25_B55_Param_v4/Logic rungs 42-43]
   // ************************************************************************************************************
   // Section of AOI that controls writing of the Device Access Locks parameter (index 12).
   // ************************************************************************************************************
   42: XIC(Device.Initial_Global_Read)XIO(Command_Being_Processed)XIO(Local_Control.11)EQU(Device.Command,43)OTL(Command_Being_Processed)MOV(0,Port_Data.Data_Transfer[0])MOV(0,Port_Data.Data_Transfer[1])BTD(Device.Write.Parameter_Access_Lock,0,Port_Data.Data_Transfer[1],0,1)BTD(Device.Write.Parameter_Access_Lock,0,Port_Data.Data_Transfer[1],0,1)BTD(Device.Write.Data_Storage_Lock,0,Port_Data.Data_Transfer[1],1,1)BTD(Device.Write.Local_Parameterization_Lock,0,Port_Data.Data_Transfer[1],2,1)BTD(Device.Write.Local_User_Interface_Lock,0,Port_Data.Data_Transfer[1],3,1)MOV(Port,Port_Data.Data_Transfer[185])MOV(0,Port_Data.Data_Transfer[187])MOV(12,Port_Data.Data_Transfer[188])MOV(2,Port_Data.Data_Transfer[189])MOV(1,Inprocess_Index)OTL(Port_Data.Port_Write.[Port])OTL(Local_Control.11);
   43: NOP();
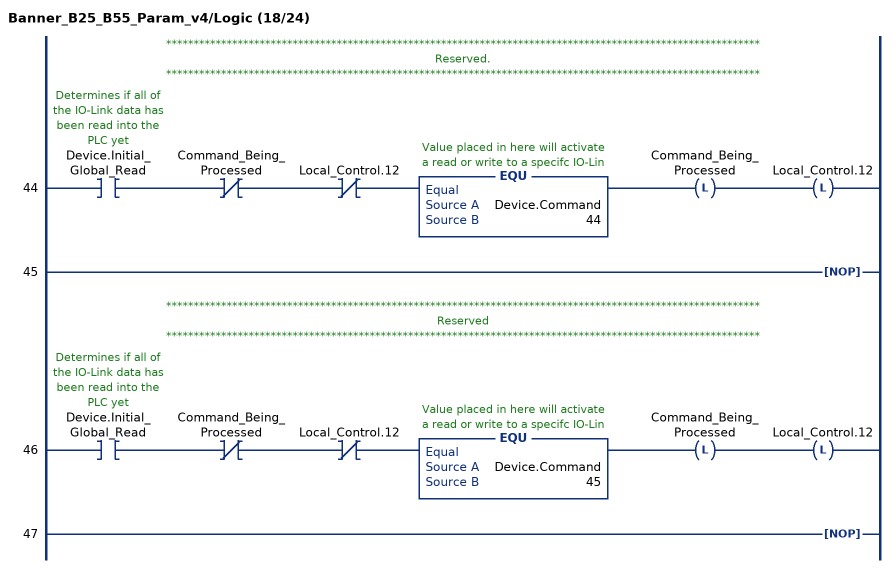
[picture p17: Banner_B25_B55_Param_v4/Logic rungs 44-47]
   // ************************************************************************************************************
   // Reserved.
   // ************************************************************************************************************
   44: XIC(Device.Initial_Global_Read)XIO(Command_Being_Processed)XIO(Local_Control.12)EQU(Device.Command,44)OTL(Command_Being_Processed)OTL(Local_Control.12);
   45: NOP();
   // ************************************************************************************************************
   // Reserved
   // ************************************************************************************************************
   46: XIC(Device.Initial_Global_Read)XIO(Command_Being_Processed)XIO(Local_Control.12)EQU(Device.Command,45)OTL(Command_Being_Processed)OTL(Local_Control.12);
   47: NOP();
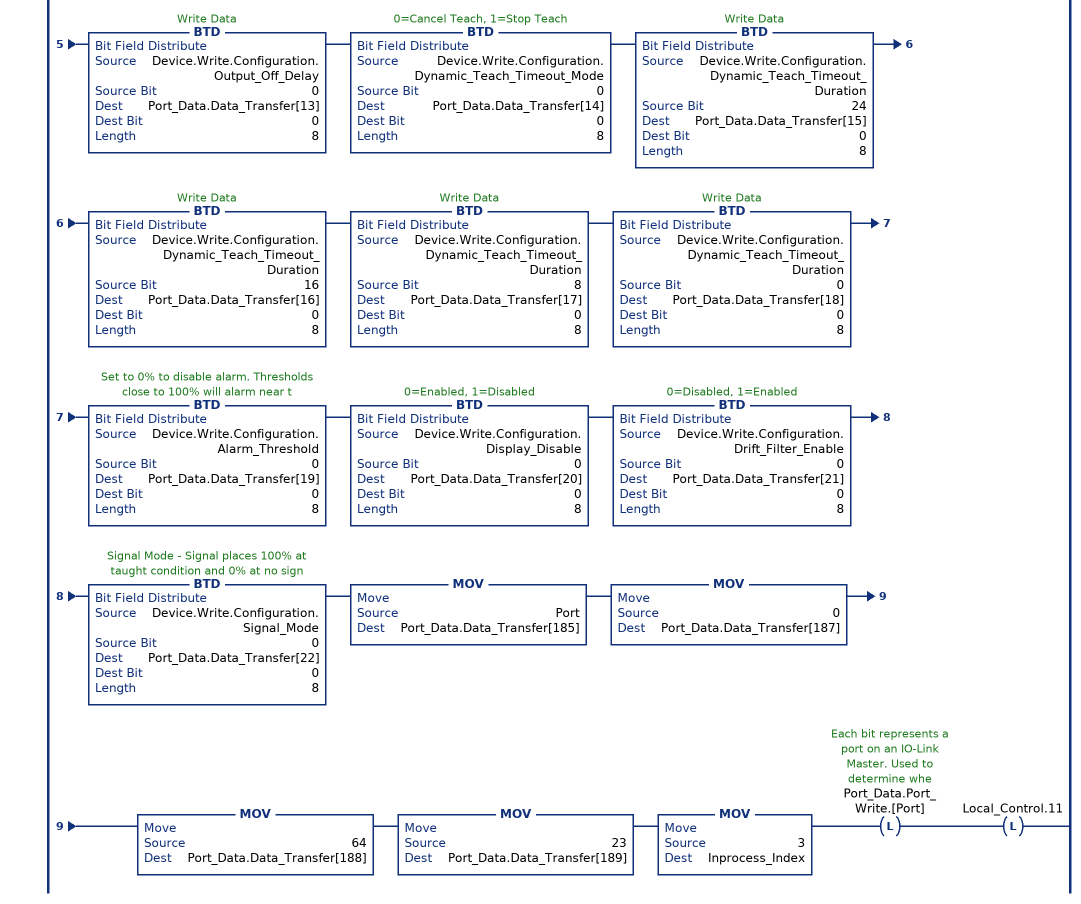
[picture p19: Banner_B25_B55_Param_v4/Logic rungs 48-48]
   // ************************************************************************************************************
   // Section of AOI that controls writing of the Configuration parameter (index 64).
   // ************************************************************************************************************
   48: XIC(Device.Initial_Global_Read)XIO(Command_Being_Processed)XIO(Local_Control.11)EQU(Device.Command,46)OTL(Command_Being_Processed)BTD(Device.Write.Configuration.Sensor_Lockout,0,Port_Data.Data_Transfer[0],0,8)BTD(Device.Write.Configuration.Sensitivity,0,Port_Data.Data_Transfer[1],0,8)BTD(Device.Write.Configuration.Pin2_Function,0,Port_Data.Data_Transfer[2],0,8)BTD(Device.Write.Configuration.Pin2_Pin4_Polarity,0,Port_Data.Data_Transfer[3],0,8)BTD(Device.Write.Configuration.Output_Logic,0,Port_Data.Data_Transfer[4],0,8)BTD(Device.Write.Configuration.Output_Delay_Mode,0,Port_Data.Data_Transfer[5],0,8)BTD(Device.Write.Configuration.Output_On_Delay,24,Port_Data.Data_Transfer[6],0,8)BTD(Device.Write.Configuration.Output_On_Delay,16,Port_Data.Data_Transfer[7],0,8)BTD(Device.Write.Configuration.Output_On_Delay,8,Port_Data.Data_Transfer[8],0,8)BTD(Device.Write.Configuration.Output_On_Delay,0,Port_Data.Data_Transfer[9],0,8)BTD(Device.Write.Configuration.Output_Off_Delay,24,Port_Data.Data_Transfer[10],0,8)BTD(Device.Write.Configuration.Output_Off_Delay,16,Port_Data.Data_Transfer[11],0,8)BTD(Device.Write.Configuration.Output_Off_Delay,8,Port_Data.Data_Transfer[12],0,8)BTD(Device.Write.Configuration.Output_Off_Delay,0,Port_Data.Data_Transfer[13],0,8)BTD(Device.Write.Configuration.Dynamic_Teach_Timeout_Mode,0,Port_Data.Data_Transfer[14],0,8)BTD(Device.Write.Configuration.Dynamic_Teach_Timeout_Duration,24,Port_Data.Data_Transfer[15],0,8)BTD(Device.Write.Configuration.Dynamic_Teach_Timeout_Duration,16,Port_Data.Data_Transfer[16],0,8)BTD(Device.Write.Configuration.Dynamic_Teach_Timeout_Duration,8,Port_Data.Data_Transfer[17],0,8)BTD(Device.Write.Configuration.Dynamic_Teach_Timeout_Duration,0,Port_Data.Data_Transfer[18],0,8)BTD(Device.Write.Configuration.Alarm_Threshold,0,Port_Data.Data_Transfer[19],0,8)BTD(Device.Write.Configuration.Display_Disable,0,Port_Data.Data_Transfer[20],0,8)BTD(Device.Write.Configuration.Drift_Filter_Enable,0,Port_Data.Data_Transfer[21],0,8)BTD(Device.Write.Configuration.Signal_Mode,0,Port_Data.Data_Transfer[22],0,8)MOV(Port,Port_Data.Data_Transfer[185])MOV(0,Port_Data.Data_Transfer[187])MOV(64,Port_Data.Data_Transfer[188])MOV(23,Port_Data.Data_Transfer[189])MOV(3,Inprocess_Index)OTL(Port_Data.Port_Write.[Port])OTL(Local_Control.11);
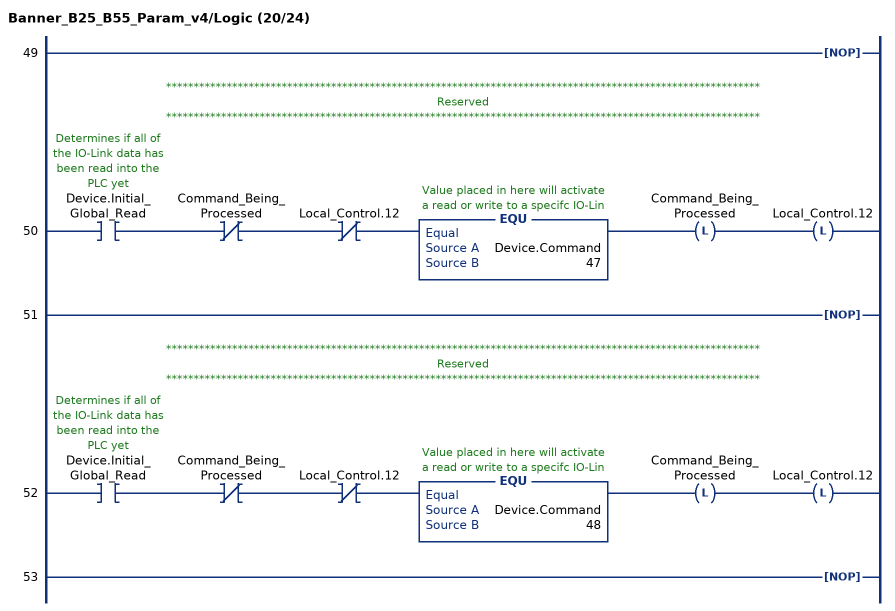
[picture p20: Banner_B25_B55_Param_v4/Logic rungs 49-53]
   49: NOP();
   // ************************************************************************************************************
   // Reserved
   // ************************************************************************************************************
   50: XIC(Device.Initial_Global_Read)XIO(Command_Being_Processed)XIO(Local_Control.12)EQU(Device.Command,47)OTL(Command_Being_Processed)OTL(Local_Control.12);
   51: NOP();
   // ************************************************************************************************************
   // Reserved
   // ************************************************************************************************************
   52: XIC(Device.Initial_Global_Read)XIO(Command_Being_Processed)XIO(Local_Control.12)EQU(Device.Command,48)OTL(Command_Being_Processed)OTL(Local_Control.12);
   53: NOP();
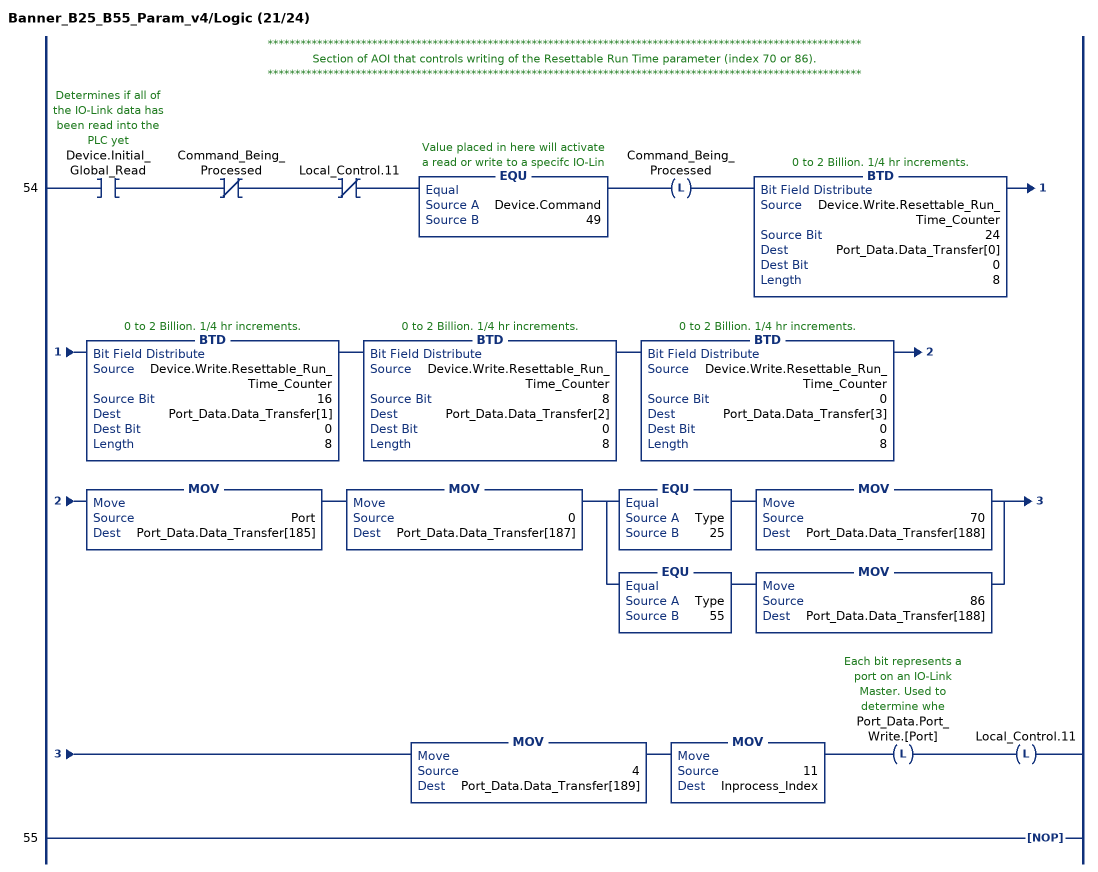
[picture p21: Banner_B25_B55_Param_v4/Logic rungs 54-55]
   // ************************************************************************************************************
   // Section of AOI that controls writing of the Resettable Run Time parameter (index 70 or 86).
   // ************************************************************************************************************
   54: XIC(Device.Initial_Global_Read)XIO(Command_Being_Processed)XIO(Local_Control.11)EQU(Device.Command,49)OTL(Command_Being_Processed)BTD(Device.Write.Resettable_Run_Time_Counter,24,Port_Data.Data_Transfer[0],0,8)BTD(Device.Write.Resettable_Run_Time_Counter,16,Port_Data.Data_Transfer[1],0,8)BTD(Device.Write.Resettable_Run_Time_Counter,8,Port_Data.Data_Transfer[2],0,8)BTD(Device.Write.Resettable_Run_Time_Counter,0,Port_Data.Data_Transfer[3],0,8)MOV(Port,Port_Data.Data_Transfer[185])MOV(0,Port_Data.Data_Transfer[187])[EQU(Type,25) MOV(70,Port_Data.Data_Transfer[188]) ,EQU(Type,55) MOV(86,Port_Data.Data_Transfer[188]) ]MOV(4,Port_Data.Data_Transfer[189])MOV(11,Inprocess_Index)OTL(Port_Data.Port_Write.[Port])OTL(Local_Control.11);
   55: NOP();
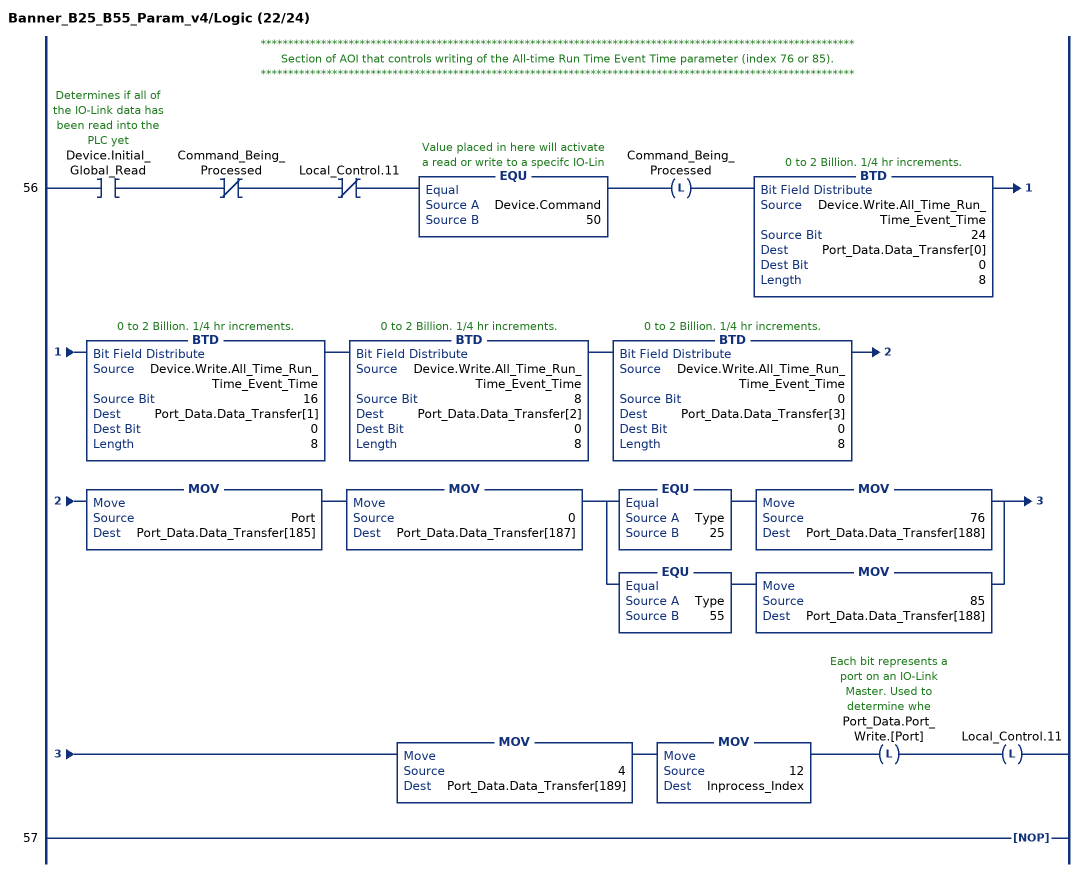
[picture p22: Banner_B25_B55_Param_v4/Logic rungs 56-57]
   // ************************************************************************************************************
   // Section of AOI that controls writing of the All-time Run Time Event Time parameter (index 76 or 85).
   // ************************************************************************************************************
   56: XIC(Device.Initial_Global_Read)XIO(Command_Being_Processed)XIO(Local_Control.11)EQU(Device.Command,50)OTL(Command_Being_Processed)BTD(Device.Write.All_Time_Run_Time_Event_Time,24,Port_Data.Data_Transfer[0],0,8)BTD(Device.Write.All_Time_Run_Time_Event_Time,16,Port_Data.Data_Transfer[1],0,8)BTD(Device.Write.All_Time_Run_Time_Event_Time,8,Port_Data.Data_Transfer[2],0,8)BTD(Device.Write.All_Time_Run_Time_Event_Time,0,Port_Data.Data_Transfer[3],0,8)MOV(Port,Port_Data.Data_Transfer[185])MOV(0,Port_Data.Data_Transfer[187])[EQU(Type,25) MOV(76,Port_Data.Data_Transfer[188]) ,EQU(Type,55) MOV(85,Port_Data.Data_Transfer[188]) ]MOV(4,Port_Data.Data_Transfer[189])MOV(12,Inprocess_Index)OTL(Port_Data.Port_Write.[Port])OTL(Local_Control.11);
   57: NOP();
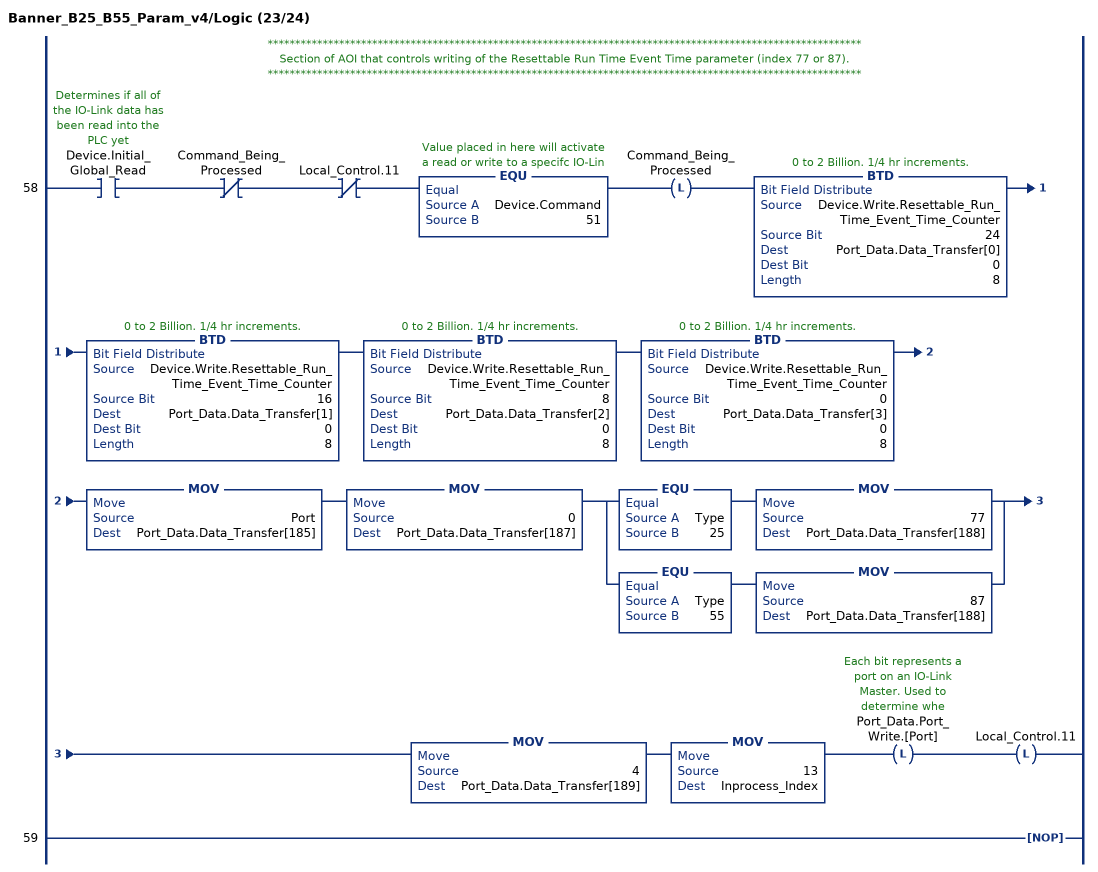
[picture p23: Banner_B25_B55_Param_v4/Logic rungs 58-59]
   // ************************************************************************************************************
   // Section of AOI that controls writing of the Resettable Run Time Event Time parameter (index 77 or 87).
   // ************************************************************************************************************
   58: XIC(Device.Initial_Global_Read)XIO(Command_Being_Processed)XIO(Local_Control.11)EQU(Device.Command,51)OTL(Command_Being_Processed)BTD(Device.Write.Resettable_Run_Time_Event_Time_Counter,24,Port_Data.Data_Transfer[0],0,8)BTD(Device.Write.Resettable_Run_Time_Event_Time_Counter,16,Port_Data.Data_Transfer[1],0,8)BTD(Device.Write.Resettable_Run_Time_Event_Time_Counter,8,Port_Data.Data_Transfer[2],0,8)BTD(Device.Write.Resettable_Run_Time_Event_Time_Counter,0,Port_Data.Data_Transfer[3],0,8)MOV(Port,Port_Data.Data_Transfer[185])MOV(0,Port_Data.Data_Transfer[187])[EQU(Type,25) MOV(77,Port_Data.Data_Transfer[188]) ,EQU(Type,55) MOV(87,Port_Data.Data_Transfer[188]) ]MOV(4,Port_Data.Data_Transfer[189])MOV(13,Inprocess_Index)OTL(Port_Data.Port_Write.[Port])OTL(Local_Control.11);
   59: NOP();
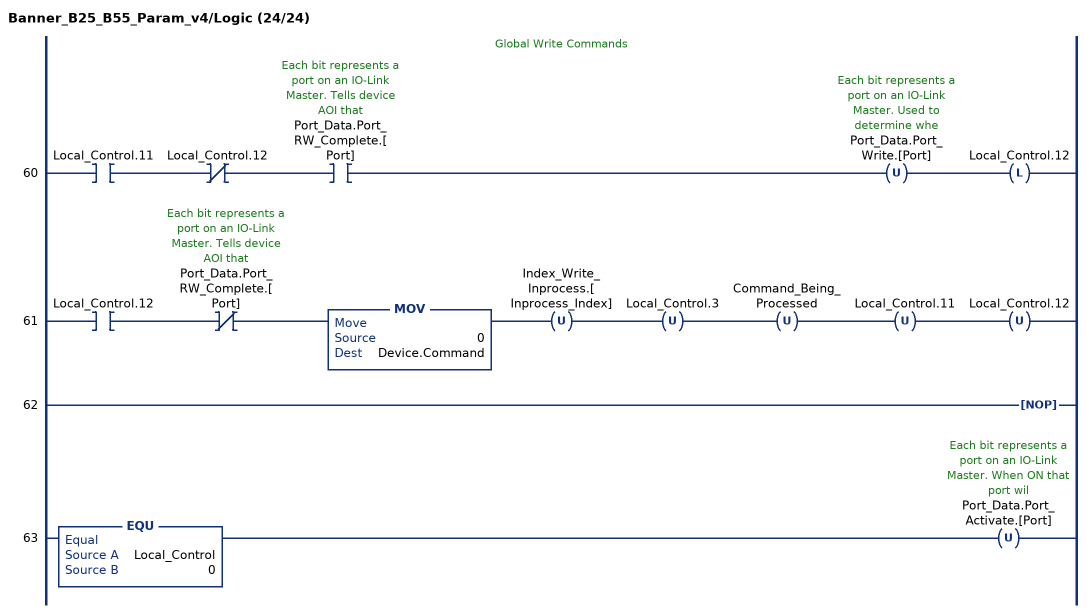
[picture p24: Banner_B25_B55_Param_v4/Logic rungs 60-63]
   // Global Write Commands
   60: XIC(Local_Control.11)XIO(Local_Control.12)XIC(Port_Data.Port_RW_Complete.[Port])OTU(Port_Data.Port_Write.[Port])OTL(Local_Control.12);
   61: XIC(Local_Control.12)XIO(Port_Data.Port_RW_Complete.[Port])MOV(0,Device.Command)OTU(Index_Write_Inprocess.[Inprocess_Index])OTU(Local_Control.3)OTU(Command_Being_Processed)OTU(Local_Control.11)OTU(Local_Control.12);
   62: NOP();
   63: EQU(Local_Control,0)OTU(Port_Data.Port_Activate.[Port]);
END_ROUTINE
END_ADD_ON_INSTRUCTION
